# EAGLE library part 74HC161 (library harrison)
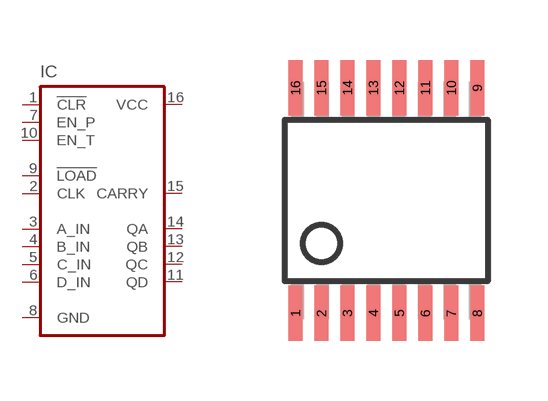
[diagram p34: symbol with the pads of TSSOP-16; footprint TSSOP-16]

Designator prefix IC

## 74HC161  [TSSOP-16]
1  !CLR!  in
2  CLK  in
3  A_IN  in
4  B_IN  in
5  C_IN  in
6  D_IN  in
7  EN_P  in
8  GND  pwr
9  !LOAD!  nc
10  EN_T  in
11  QD  out
12  QC  out
13  QB  out
14  QA  out
15  CARRY  out
16  VCC  pwr

## Footprint TSSOP-16 (pad centres in mm)
smd 0.348 x 1.397: 1 -2.273,-2.814; 2 -1.623,-2.815; 3 -0.973,-2.815; 4 -0.323,-2.815; 5 0.327,-2.815; 6 0.977,-2.815; 7 1.627,-2.815; 8 2.277,-2.815; 9 2.277,2.825; 10 1.627,2.825; 11 0.977,2.825; 12 0.327,2.825; 13 -0.323,2.825; 14 -0.973,2.825; 15 -1.623,2.825; 16 -2.273,2.825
